| ZCH_DESIGN_SPEC   IBIS MODEL   |
[IBIS Ver]   3.2
[Comment Char]   |_char
[File Name]   sprm497.ibs
[File Rev]   1.0
[Date]   March 10, 2010
[Source]   TI
[Disclaimer]   Please be aware that in the absence of a written agreement
|   Texas Instruments (TI) assumes no liability for:   |
|   (1) The accuracy of the IBIS models provided to your company   |
|   (2) The proper functioning of these Models in your design   |
|   or for any resulting applications   |
|   (3) Infringement of patents, copyrights or intellectual   |
|   property rights resulting from your use of these   |
|   models.   |
|   TI provides IBIS Models as a service to our customers and   |
|   therefore reserves the right to limit distribution of the   |
|   Models.   |
[Copyright]   Property of Texas Instruments Incorporated.
|   Unauthorized reproduction and/or distribution is strictly.   |
|   prohibited.   |
|   This product is protected under copyright law and trade   |
|   secret law as an unpublished work.   |
|   Created 2003,(C) Copyright 1999-2003,   |
|   Texas Instruments Incorporated. All Rights Reserved.   |
|   These commodities are under the U.S. Government   |
|   distribution license control. As such, they are not to be   |
|   re-exported without the prior approval of the U.S.   |
|   Department of Commerce.   |
[Notes]
|***************************  Package Models  ************************************|
| Component   C5515_ZCH   |
[Component]   C5515_ZCH
[Manufacturer]   Texas Instruments
[Package]
| variable   typ   min   max
R_pkg   1.65496e-001  2.14143e-002  2.82384e-001
L_pkg   2.60932e-009  7.69280e-011  4.87010e-009
C_pkg   1.03072e-012  5.05112e-013  9.54198e-012
[Pin]   signal_name   model_name   R_pin   L_pin   C_pin
B2   EM_A0   BC3340CTSCHY   2.10E-01   2.89E-09   5.81E-13
B3   EM_CS0   BC3340CTSCHY   2.18E-01   2.72E-09   6.77E-13
B1   EM_BA1   BC3340CTSCHY   1.69E-01   3.26E-09   8.03E-13
A1   EM_BA0   BC3340CTSCHY   2.33E-01   3.78E-09   6.59E-13
C2   EM_A1   BC3340CTSCHY   1.85E-01   2.63E-09   6.84E-13
C1   EM_A4   BC3340CTSCHY   1.67E-01   3.20E-09   7.67E-13
D3   EM_D10   BC3340CTSCHY   2.47E-01   3.77E-09   9.20E-13
L2   EM_A10   BC3340CTSCHY   1.18E-01   1.93E-09   8.47E-13
L3   EM_D12   BC3340CTSCHY   2.03E-01   2.77E-09   7.35E-13
K3   EM_D14   BC3340CTSCHY   1.95E-01   2.55E-09   7.29E-13
L4   EM_D4   BC3340CTSCHY   1.18E-01   1.70E-09   9.84E-13
L1   EM_A13   BC3340CTSCHY   2.07E-01   3.17E-09   7.07E-13
K2   EM_A11_ALE   BC3340CTSCHY   1.34E-01   2.33E-09   7.16E-13
K4   EM_D13   BC3340CTSCHY   1.10E-01   1.50E-09   7.10E-13
K5   EM_D6   BC3340CTSCHY   1.30E-01   2.01E-09   1.13E-12
K1   EM_A12_CLE   BC3340CTSCHY   2.00E-01   3.12E-09   6.76E-13
M3   EM_SDCLK   BC3340CTSCHY   2.02E-01   2.70E-09   8.45E-13
M1   EM_A14   BC3340CTSCHY   2.06E-01   2.89E-09   5.82E-13
M2   EM_D5   BC3340CTSCHY   1.24E-01   2.10E-09   1.01E-12
N2   EM_SDCKE   BC3340CTSCHY   1.74E-01   3.20E-09   9.99E-13
P1   EM_DQM1   BC3340CTSCHY   2.02E-01   3.74E-09   9.11E-13
E3   EM_D8   BC3340CTSCHY   2.36E-01   3.60E-09   8.20E-13
F4   EM_D9   BC3340CTSCHY   1.29E-01   1.81E-09   9.00E-13
E1   EM_A2   BC3340CTSCHY   1.91E-01   2.92E-09   7.13E-13
F3   EM_D2   BC3340CTSCHY   1.68E-01   2.02E-09   8.37E-13
F1   EM_A6   BC3340CTSCHY   1.86E-01   2.87E-09   6.26E-13
G1   EM_WAIT4   BC3340CTSCHY   1.46E-01   2.80E-09   7.40E-13
G3   EM_D0   BC3340CTSCHY   1.52E-01   2.15E-09   1.06E-12
H3   EM_D7   BC3340CTSCHY   9.97E-02   1.51E-09   6.15E-13
J4   EM_D15   BC3340CTSCHY   2.11E-01   3.00E-09   8.75E-13
J2   EM_A9   BC3340CTSCHY   1.65E-01   2.08E-09   8.02E-13
D2   EM_A3   BC3340CTSCHY   1.33E-01   2.35E-09   7.63E-13
D1   EM_A5   BC3340CTSCHY   2.00E-01   3.07E-09   7.12E-13
E4   EM_OE   BC3340CTSCHY   1.15E-01   1.51E-09   9.68E-13
H2   EM_A7   BC3340CTSCHY   2.13E-01   3.13E-09   6.67E-13
H1   EM_WE   BC3340CTSCHY   1.46E-01   2.87E-09   6.78E-13
J1   EM_A8   BC3340CTSCHY   1.47E-01   2.82E-09   7.20E-13
K6   EM_WAIT3   BC3340CTSCHY   2.33E-01   3.46E-09   1.30E-12
C3   EM_CS4   BC3340CTSCHY   2.23E-01   2.73E-09   7.77E-13
A3   EM_CS5   BC3340CTSCHY   2.10E-01   3.78E-09   8.09E-13
B4   EM_SDCAS   BC3340CTSCHY   2.79E-01   4.04E-09   8.65E-13
H4   EM_WAIT5   BC3340CTSCHY   1.84E-01   2.36E-09   9.32E-13
B6   EM_R_W   BC3340CTSCHY   1.41E-01   2.06E-09   7.85E-13
E5   EM_D1   BC3340CTSCHY   1.32E-01   2.27E-09   1.25E-12
D5   EM_WAIT2   BC3340CTSCHY   2.73E-01   3.58E-09   1.15E-12
C5   EM_CS2   BC3340CTSCHY   1.40E-01   1.77E-09   8.20E-13
C4   EM_D11   BC3340CTSCHY   2.39E-01   2.98E-09   8.05E-13
B5   EM_DQM0   BC3340CTSCHY   2.45E-01   3.21E-09   7.61E-13
D4   EM_D3   BC3340CTSCHY   1.76E-01   2.40E-09   1.01E-12
M4   EM_CS3   BC3340CTSCHY   1.33E-01   1.97E-09   8.96E-13
A6   EM_SDRAS   BC3340CTSCHY   2.11E-01   2.91E-09   6.68E-13
A4   EM_CS1   BC3340CTSCHY   1.74E-01   2.97E-09   7.26E-13
N1   EM_A15_GP21   BC3340CTSCHYPD 2.39E-01   3.42E-09   5.97E-13
E2   EM_A16_GP22   BC3340CTSCHYPD 1.28E-01   2.26E-09   8.17E-13
F2   EM_A17_GP23   BC3340CTSCHYPD 1.04E-01   1.77E-09   7.80E-13
G4   EM_A19_GP25   BC3340CTSCHYPD 2.06E-01   2.82E-09   7.99E-13
G2   EM_A18_GP24   BC3340CTSCHYPD 2.10E-01   3.09E-09   6.98E-13
J3   EM_A20_GP26   BC3340CTSCHYPD 1.62E-01   2.58E-09   1.25E-12
N4   LCD_CS1_EN1_SPI_CS1   BC3350CTHY   1.61E-01   2.21E-09   5.99E-13
N5   LCD_RS_SPI_CS3   BC3350CTHY   1.14E-01   2.01E-09   7.53E-13
P4   LCD_CS0_E0_SPI_CS0   BC3350CTHY   1.40E-01   2.87E-09   7.71E-13
P5   LCD_RW_WRB_SPI_CS2   BC3350CTHY   1.77E-01   2.90E-09   7.33E-13
P6   LCDD0_SPI_RX   BC3350CTHY   1.68E-01   2.77E-09   6.88E-13
N6   LCDD1_SPI_TX   BC3350CTHY   1.10E-01   2.01E-09   7.72E-13
P7   LCDD2_GP12   BC3350CTHYPD   1.24E-01   2.50E-09   7.10E-13
N11   LCDD10_I2S2_RX_GP20_SPI_RX   BC3350CTHYPD   1.52E-01   2.25E-09   6.62E-13
M12   MMC1_D1_I2S1_RX_GP9   BC3350CTHYPD   2.23E-01   3.66E-09   7.57E-13
M11   MMC0_CMD_I2S0_FS_GP1   BC3350CTHYPD   1.09E-01   1.70E-09   7.27E-13
P11   LCDD9_I2S2_FS_GP19_SPI_CS0   BC3350CTHYPD   1.36E-01   2.87E-09   7.14E-13
N12   LCDD12_UARTRTS_GP28_I2S3_CLK   BC3350CTHYPD   1.77E-01   3.41E-09   7.41E-13
P12   LCDD11_I2S2_DX_GP27_SPI_TX   BC3350CTHYPD   1.63E-01   2.44E-09   5.05E-13
P13   LCDD13_UARTCTS_GP29_I2S3_FS   BC3350CTHYPD   2.10E-01   3.20E-09   5.66E-13
N13   LCDD14_UARTRXD_GP30_I2S3_RX   BC3350CTHYPD   1.40E-01   2.70E-09   7.84E-13
P14   LCDD15_UARTTXD_GP31_I2S3_DX   BC3350CTHYPD   1.51E-01   3.07E-09   6.72E-13
N7   LCDD3_GP13   BC3350CTHYPD   1.40E-01   1.97E-09   6.29E-13
N8   LCDD4_GP14   BC3350CTHYPD   1.41E-01   2.04E-09   7.00E-13
N9   LCDD6_GP16   BC3350CTHYPD   1.26E-01   2.21E-09   7.81E-13
L9   MMC0_D0_I2S0_DX_GP2   BC3350CTHYPD   1.32E-01   2.04E-09   1.24E-12
P9   LCDD5_GP15   BC3350CTHYPD   1.66E-01   2.73E-09   5.96E-13
M10   MMC0_D1_I2S0_RX_GP3   BC3350CTHYPD   2.12E-01   3.53E-09   8.62E-13
L10   MMC0_CLK_I2S0_CLK_GP0   BC3350CTHYPD   1.21E-01   2.10E-09   1.26E-12
P10   LCDD7_GP17   BC3350CTHYPD   1.31E-01   2.64E-09   8.11E-13
L11   MMC0_D3_GP5   BC3350CTHYPD   1.94E-01   2.78E-09   1.14E-12
N10   LCDD8_I2S2_CLK_GP18_SPI_CLK   BC3350CTHYPD   1.15E-01   2.40E-09   8.58E-13
L12   MMC0_D2_GP4   BC3350CTHYPD   2.45E-01   3.56E-09   7.75E-13
L13   MMC1_D3_GP11   BC3350CTHYPD   1.36E-01   2.30E-09   6.70E-13
M14   MMC1_D0_I2S1_DX_GP8   BC3350CTHYPD   1.64E-01   3.07E-09   5.83E-13
M13   MMC1_CLK_I2S1_CLK_GP6   BC3350CTHYPD   1.83E-01   2.54E-09   5.51E-13
L14   MMC1_CMD_I2S1_FS_GP7   BC3350CTHYPD   1.90E-01   3.10E-09   5.39E-13
K14   MMC1_D2_GP10   BC3350CTHYPD   1.58E-01   3.08E-09   6.45E-13
L6   EMU0   BC3350CTHYPU   9.20E-02   1.26E-09   9.54E-13
M5   EMU1   BC3350CTHYPU   1.59E-01   2.01E-09   7.80E-13
E8   WAKEUP   BI2C33S   2.07E-01   3.19E-09   1.42E-12
C7   CLK_SEL   IC33THY   2.03E-01   2.65E-09   1.22E-12
A8   CLKIN   IC33THY   1.85E-01   3.14E-09   7.97E-13
M9   TRST   IC33THYPD   1.44E-01   1.93E-09   8.03E-13
D6   RESET   IC33THYPU   1.73E-01   2.47E-09   1.33E-12
C6   INT0   IC33THYPU   2.40E-01   3.00E-09   1.13E-12
E7   INT1   IC33THYPU   2.82E-01   4.11E-09   1.56E-12
M6   TCK   IC33THYPU   1.49E-01   1.90E-09   8.84E-13
L7   TDI   IC33THYPU   1.09E-01   1.70E-09   1.08E-12
L8   TMS   IC33THYPU   1.66E-01   2.15E-09   9.72E-13
A7   CLKOUT   OC3340CTSC   2.10E-01   3.01E-09   6.50E-13
D8   RTCCLKOUT   OC3350CT   1.82E-01   2.62E-09   1.34E-12
N3   LCD_EN_RDB_SPI_CLK   OC3350CT   1.66E-01   3.02E-09   8.89E-13
M8   XF   OC3350CT   8.38E-02   1.35E-09   8.20E-13
M7   TDO   OC3350CT   1.69E-01   2.20E-09   9.82E-13
B7   SCL   BI2C33T   8.34E-02   1.45E-09   6.42E-13
B8   SDA   BI2C33T   2.37E-01   3.53E-09   7.21E-13
|[End Package Model]
|***********************************  Buffer Models  ***************************
|   Component BC3340CTSCHY
[Component]   BC3340CTSCHY
[Manufacturer]   Texas Instruments
[Package]
|  variable   typ   min   max
R_pkg   0   0   0
L_pkg   0   0   0
C_pkg   0   0   0
[Pin]   signal_name   model_name   R_pin   L_pin   C_pin
VSS   VSS   GND
VDDS   VDDS   POWER
PAD   PAD   BC3340CTSCHY
[Model Selector] BC3340CTSCHY
SR0_VDD_SR1_VDD_3P3  Cell operated at 3.3(nom)
|SR0_VDD_SR1_VDD_3P3CELL OPERATING IN FAST MODE
SR0_VSS_SR1_VSS_3P3  Cell operated at 3.3(nom)
|   Component BC3340CTSCHYPD
[Component]   BC3340CTSCHYPD
[Manufacturer]   Texas Instruments
[Package]
|  variable   typ   min   max
R_pkg   0   0   0
L_pkg   0   0   0
C_pkg   0   0   0
[Pin]   signal_name   model_name   R_pin   L_pin   C_pin
VSS   VSS   GND
VDDS   VDDS   POWER
PAD   PAD   BC3340CTSCHYPD
[Model Selector] BC3340CTSCHYPD
S_SR1_VSS_PD_OFF_3P3  Cell operated at 3.3(nom)
|SR0_VSS_SR1_VSS_PD_OFF_3P3CELL OPERATING IN SLOW MODE WITH PULLDOWN OFF
SS_SR1_VSS_PD_ON_3P3  Cell operated at 3.3(nom)
|SR0_VSS_SR1_VSS_PD_ON_3P3CELL OPERATING IN SLOW MODE AT 100UA WITH PULLDOW
|N ON
DD_SR1_VDD_PD_ON_3P3  Cell operated at 3.3(nom)
|SR0_VDD_SR1_VDD_PD_ON_3P3CELL OPERATING IN FAST MODE AT 100UA WITH PULLDOW
|N ON
D_SR1_VDD_PD_OFF_3P3  Cell operated at 3.3(nom)
|   Component BC3350CTHYPD
[Component]   BC3350CTHYPD
[Manufacturer]   Texas Instruments
[Package]
|  variable   typ   min   max
R_pkg   0   0   0
L_pkg   0   0   0
C_pkg   0   0   0
[Pin]   signal_name   model_name   R_pin   L_pin   C_pin
VSS   VSS   GND
VDDS   VDDS   POWER
PAD   PAD   BC3350CTHYPD
[Model Selector] BC3350CTHYPD
PULLDOWN_ON_COM  Cell operated at 3.3(nom) COM Temp PULLDOWN_ON
PULLDOWN_OFF_COM  Cell operated at 3.3(nom) COM Temp PULLDOWN_OFF
PULLDOWN_ON_IND  Cell operated at 3.3(nom) IND Temp PULLDOWN_ON
PULLDOWN_OFF_IND  Cell operated at 3.3(nom) IND Temp PULLDOWN_OFF
|   Component BI2C33S
[Component]   BI2C33S
[Manufacturer]   Texas Instruments
[Package]
|  variable   typ   min   max
R_pkg   0   0   0
L_pkg   0   0   0
C_pkg   0   0   0
[Pin]   signal_name   model_name   R_pin   L_pin   C_pin
VSS   VSS   GND
VDDS   VDDS   POWER
PAD   PAD   BI2C33S
|   Component IC33THYPD
[Component]   IC33THYPD
[Manufacturer]   Texas Instruments
[Package]
|  variable   typ   min   max
R_pkg   0   0   0
L_pkg   0   0   0
C_pkg   0   0   0
[Pin]   signal_name   model_name   R_pin   L_pin   C_pin
VSS   VSS   GND
VDDS   VDDS   POWER
PAD   PAD   IC33THYPD
[Model Selector] IC33THYPD
PULLDOWN_ON_COMM  Cell operated at 3.3(nom) COM Temp PULLDOWN_ON
PULLDOWN_OFF_COMM  Cell operated at 3.3(nom) COM Temp PULLDOWN_OFF
PULLDOWN_ON_INDD  Cell operated at 3.3(nom) IND Temp PULLDOWN_ON
PULLDOWN_OFF_INDD  Cell operated at 3.3(nom) IND Temp PULLDOWN_OFF
|   Component IC33THYPU
[Component]   IC33THYPU
[Manufacturer]   Texas Instruments
[Package]
|  variable   typ   min   max
R_pkg   0   0   0
L_pkg   0   0   0
C_pkg   0   0   0
[Pin]   signal_name   model_name   R_pin   L_pin   C_pin
VSS   VSS   GND
VDDS   VDDS   POWER
PAD   PAD   IC33THYPU
[Model Selector] IC33THYPU
PULLUP_ON_COM  Cell operated at 3.3(nom) COM Temp PULLUP_ON
PULLUP_OFF_COM  Cell operated at 3.3(nom) COM Temp PULLUP_OFF
PULLUP_ON_IND  Cell operated at 3.3(nom) IND Temp PULLUP_ON
PULLUP_OFF_IND  Cell operated at 3.3(nom) IND Temp PULLUP_OFF
|   Component BC3350CTHYPU
[Component]   BC3350CTHYPU
[Manufacturer]   Texas Instruments
[Package]
|  variable   typ   min   max
R_pkg   0   0   0
L_pkg   0   0   0
C_pkg   0   0   0
[Pin]   signal_name   model_name   R_pin   L_pin   C_pin
VSS   VSS   GND
VDDS   VDDS   POWER
PAD   PAD   BC3350CTHYPU
[Model Selector] BC3350CTHYPU
350CTHYPU_PU_ON_2P75  Cell operated at 2.75(nom)
|BC3350CTHYPU_PU_ON_2P75; CELL IN PULLUP MODE WITH PI=0
50CTHYPU_PU_OFF_2P75  Cell operated at 2.75(nom)
|BC3350CTHYPU_PU_OFF_2P75; CELL IN NORMAL MODE WITH PULLUP DISABLED
3350CTHYPU_PU_ON_1P8  Cell operated at 1.8(nom)
|BC3350CTHYPU_PU_ON_1P8; CELL IN PULLUP MODE WITH PI=0
350CTHYPU_PU_OFF_1P8  Cell operated at 1.8(nom)
|BC3350CTHYPU_PU_OFF_1P8; CELL IN NORMAL MODE WITH PULLUP DISABLED
3350CTHYPU_PU_ON_2P5  Cell operated at 2.5(nom)
|BC3350CTHYPU_PU_ON_2P5; CELL IN PULLUP MODE WITH PI=0
350CTHYPU_PU_OFF_2P5  Cell operated at 2.5(nom)
|BC3350CTHYPU_PU_OFF_2P5; CELL IN NORMAL MODE WITH PULLUP DISABLED
3350CTHYPU_PU_ON_3P3  Cell operated at 3.3(nom)
|BC3350CTHYPU_PU_ON_3P3; CELL IN PULLUP MODE WITH PI=0
350CTHYPU_PU_OFF_3P3  Cell operated at 3.3(nom)
|   Component IC33THY
[Component]   IC33THY
[Manufacturer]   Texas Instruments
[Package]
|  variable   typ   min   max
R_pkg   0   0   0
L_pkg   0   0   0
C_pkg   0   0   0
[Pin]   signal_name   model_name   R_pin   L_pin   C_pin
VDDS   VDDS   POWER
VSS   VSS   GND
PAD   PAD   IC33THY
[Model Selector] IC33THY
IC33THY_2P75  Cell operated at 2.75(nom)
|IC33THY_2P75;
IC33THY_1P8  Cell operated at 1.8(nom)
|IC33THY_1P8;
IC33THY_2P5  Cell operated at 2.5(nom)
|IC33THY_2P5;
IC33THY_3P3  Cell operated at 3.3(nom)
|   Component OC3340CTSC
[Component]   OC3340CTSC
[Manufacturer]   Texas Instruments
[Package]
|  variable   typ   min   max
R_pkg   0   0   0
L_pkg   0   0   0
C_pkg   0   0   0
[Pin]   signal_name   model_name   R_pin   L_pin   C_pin
VSS   VSS   GND
VDDS   VDDS   POWER
PAD   PAD   OC3340CTSC
[Model Selector] OC3340CTSC
SR0_VDD_SR1_VDD_3P3b  Cell operated at 3.3(nom)
|SR0_VDD_SR1_VDD_3P3b CELL OPERATING IN FAST MODE
SR0_VSS_SR1_VSS_3P3b  Cell operated at 3.3(nom)
|   Component BI2C33T
[Component]   BI2C33T
[Manufacturer]   Texas Instruments
[Package]
|  variable   typ   min   max
R_pkg   0   0   0
L_pkg   0   0   0
C_pkg   0   0   0
[Pin]   signal_name   model_name   R_pin   L_pin   C_pin
VSS   VSS   GND
VDDS   VDDS   POWER
PAD   PAD   BI2C33T
|   Component BC3350CTHY
[Component]   BC3350CTHY
[Manufacturer]   Texas Instruments
[Package]
|  variable   typ   min   max
R_pkg   0   0   0
L_pkg   0   0   0
C_pkg   0   0   0
[Pin]   signal_name   model_name   R_pin   L_pin   C_pin
VSS   VSS   GND
VDDS   VDDS   POWER
PAD   PAD   BC3350CTHY
[Model Selector] BC3350CTHY
BC3350CTHY_2P75  Cell operated at 2.75(nom)
|CELL IN NORMAL MODE AT 2.75 NOM VOLTAGE
BC3350CTHY_1P8  Cell operated at 1.8(nom)
|CELL IN NORMAL MODE AT 1.8 NOM VOLTAGE
BC3350CTHY_2P5  Cell operated at 2.5(nom)
|CELL IN NORMAL MODE AT 2.5 NOM VOLTAGE
BC3350CTHY_3P3  Cell operated at 3.3(nom)
|   Component OC3350CT
[Component]   OC3350CT
[Manufacturer]   Texas Instruments
[Package]
|  variable   typ   min   max
R_pkg   0   0   0
L_pkg   0   0   0
C_pkg   0   0   0
[Pin]   signal_name   model_name   R_pin   L_pin   C_pin
VSS   VSS   GND
VDDS   VDDS   POWER
PAD   PAD   OC3350CT
[Model Selector] OC3350CT
OC3350CT_2P75  Cell operated at 2.75(nom)
|CELL IN NORMAL MODE AT 2.75 NOM VOLTAGE
OC3350CT_1P8  Cell operated at 1.8(nom)
|CELL IN NORMAL MODE AT 1.8 NOM VOLTAGE
OC3350CT_2P5  Cell operated at 2.5(nom)
|CELL IN NORMAL MODE AT 2.5 NOM VOLTAGE
OC3350CT_3P3  Cell operated at 3.3(nom)
| Models and submodels in the file (42): SR0_VDD_SR1_VDD_3P3 (I/O), SR0_VSS_SR1_VSS_3P3 (I/O), S_SR1_VSS_PD_OFF_3P3 (I/O), SS_SR1_VSS_PD_ON_3P3 (I/O), DD_SR1_VDD_PD_ON_3P3 (I/O), D_SR1_VDD_PD_OFF_3P3 (I/O), PULLDOWN_ON_COM (I/O), PULLDOWN_OFF_COM (I/O), PULLDOWN_ON_IND (I/O), PULLDOWN_OFF_IND (I/O), BI2C33S (I/O_open_drain), PULLDOWN_ON_COMM (Input), PULLDOWN_OFF_COMM (Input), PULLDOWN_ON_INDD (Input), PULLDOWN_OFF_INDD (Input), PULLUP_ON_COM (Input), PULLUP_OFF_COM (Input), PULLUP_ON_IND (Input), PULLUP_OFF_IND (Input), 350CTHYPU_PU_ON_2P75 (I/O), 50CTHYPU_PU_OFF_2P75 (I/O), 3350CTHYPU_PU_ON_1P8 (I/O), 350CTHYPU_PU_OFF_1P8 (I/O), 3350CTHYPU_PU_ON_2P5 (I/O), 350CTHYPU_PU_OFF_2P5 (I/O), 3350CTHYPU_PU_ON_3P3 (I/O), 350CTHYPU_PU_OFF_3P3 (I/O), IC33THY_2P75 (Input), IC33THY_1P8 (Input), IC33THY_2P5 (Input), IC33THY_3P3 (Input), SR0_VDD_SR1_VDD_3P3b (3-state), SR0_VSS_SR1_VSS_3P3b (3-state), BI2C33T (I/O_open_drain), BC3350CTHY_2P75 (I/O), BC3350CTHY_1P8 (I/O), BC3350CTHY_2P5 (I/O), BC3350CTHY_3P3 (I/O), OC3350CT_2P75 (3-state), OC3350CT_1P8 (3-state), OC3350CT_2P5 (3-state), OC3350CT_3P3 (3-state)
